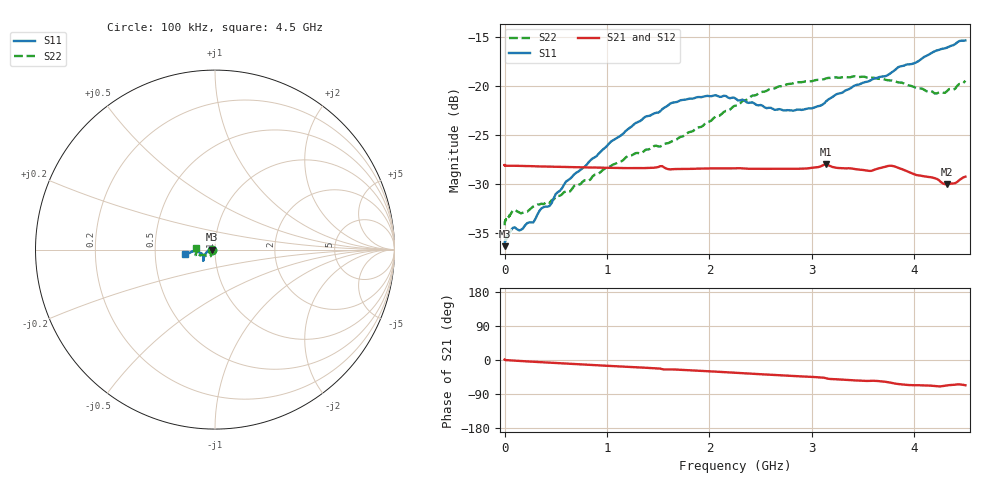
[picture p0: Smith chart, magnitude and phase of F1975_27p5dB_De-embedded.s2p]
! Integrated Device Technology
! Corporate Headquarters
! 6024 Silver Creek Valley Road
! San Jose, CA 95138  USA
! Phone:  1-408-284-8200
! Toll Free:  1-800-223-1366
! Webpage:  http://www.idt.com/
! Timing and RF Division
! 515 Groton Road, Suite 102
! Westford, MA 01886-6024
! Device:  F1975
! Description: 6-bit, 75 ohm, 0.5 dB Digital Step Attenuator
! Frequency:  5.0 MHz -  3.00 GHz
! Package:  4x4 mm QFN Plastic Package: 20 pin
! Ports:  2 RF, 11 DC
!  Pin  1  = D5 (16 dB)
!  Pin  2  = RF1  =  Port 1
!  Pin  3  = Serial Data In (DATA)
!  Pin  4  = Serial Clock (CLK)
!  Pin  5  = Serial Latch Enable (LE)
!  Pin  6  = VDD
!  Pin  7  = NC
!  Pin  8  = NC
!  Pin  9  = NC
!  Pin 10  = GND
!  Pin 11  = GND
!  Pin 12  = NC
!  Pin 13  = VMODE
!  Pin 14  = RF2  =  Port 2
!  Pin 15  = D4 (8 dB)
!  Pin 16  = D3 (4 dB)
!  Pin 17  = D2 (2 dB)
!  Pin 18  = NC
!  Pin 19  = D1 (1 dB)
!  Pin 20  = D0 (0.5 dB)
! State:  55
! Atten State:  27.5 dB
! Voltage:  +3.30 Volts
! Current:  0.562 mA
! Data:  The device was measured on a F1975 evaluation board which has
!  individual transmission lines to the RF pins.  Data was collected
!  using a calibrated network analyzer.  The evaluation board was
!  de-embedded using Automatic Fixture Removal (AFR).
!  The reference plane is the edge of the package pin.
! Misc:
!  Action Tracker AT0415
! Date Measured:  2018-02-08
! Date:  2018-03-26  MJV
! Note:
!  Integrated Device Technology supplies this data as a sample of measured
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# GHz S dB R 75
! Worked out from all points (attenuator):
!   291 points, 100 kHz to 4.5 GHz, reference 75 ohm
!   highest |S21| = -28.00 dB at 3.14 GHz (marker M1); lowest = -30.0 dB at 4.32 GHz (marker M2)
!   lowest |S11| = -36.3 dB at 100 kHz (marker M3), VSWR 1.03, Z = 72.7 - j0.00281 ohm
!   |S11| at or under -10 dB: start of sweep to end of sweep
!   |S22| runs from -34.2 to -19.0 dB; largest |S21 - S12| = 0.00014
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0.0001  -36.34 -179.9  -28.07 1.2  -28.07 1.2  -34.20 -178.8
0.004  -35.78 -178.2  -28.12 0.6  -28.14 0.6  -33.84 -178.1
0.08  -34.48 -176.3  -28.14 -1.4  -28.14 -1.4  -32.70 -169.1
0.16  -34.67 -177.6  -28.16 -2.7  -28.16 -2.7  -32.99 -159.0
0.28  -33.92 179.5  -28.19 -4.6  -28.19 -4.6  -32.30 -151.1
0.36  -32.49 179.4  -28.21 -5.9  -28.21 -5.9  -32.00 -143.3
0.44  -32.24 -179.8  -28.23 -7.1  -28.23 -7.1  -31.91 -137.4
0.6  -29.75 -176.3  -28.27 -9.5  -28.27 -9.4  -30.75 -131.5
0.76  -28.40 -169.6  -28.31 -11.8  -28.30 -11.8  -29.79 -127.8
1.28  -23.79 -152.9  -28.38 -19.1  -28.38 -19.1  -26.85 -123.7
1.52  -22.59 -144.7  -28.19 -22.7  -28.19 -22.8  -26.18 -130.4
1.62  -21.79 -142.9  -28.51 -24.8  -28.51 -24.8  -25.73 -133.8
1.88  -21.15 -138.9  -28.44 -27.8  -28.44 -27.8  -24.26 -146.5
2.26  -21.33 -137.8  -28.41 -33.8  -28.40 -33.8  -22.01 -157.6
2.64  -22.45 -147.1  -28.45 -39.6  -28.45 -39.6  -20.25 -159.0
3.02  -22.23 -163.6  -28.33 -44.9  -28.32 -44.9  -19.47 -159.9
3.14  -21.57 -166.4  -28.00 -48.3  -28.00 -48.3  -19.24 -160.3
3.56  -19.52 -176.9  -28.67 -55.2  -28.67 -55.2  -19.20 -165.9
3.76  -18.78 -175.6  -28.14 -59.4  -28.14 -59.3  -19.45 -169.6
4.2  -16.48 -172.4  -29.41 -68.5  -29.40 -68.5  -20.77 178.9
4.32  -16.11 -172.0  -30.04 -67.1  -30.04 -67.1  -20.54 176.5
4.5  -15.37 -171.9  -29.26 -66.7  -29.25 -66.7  -19.48 174.0
